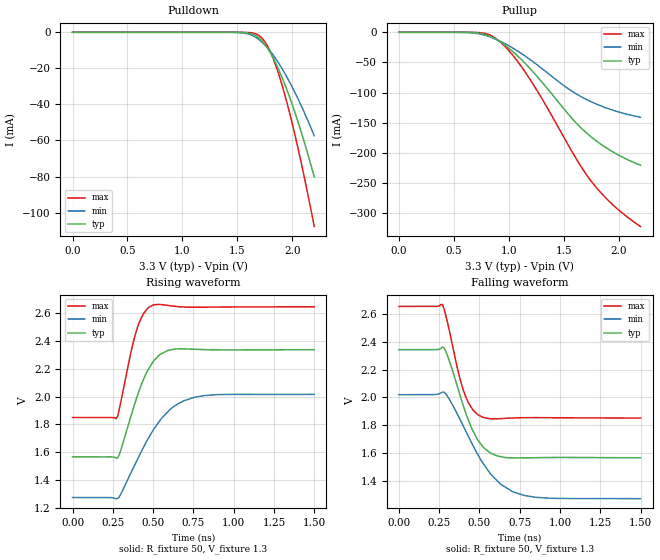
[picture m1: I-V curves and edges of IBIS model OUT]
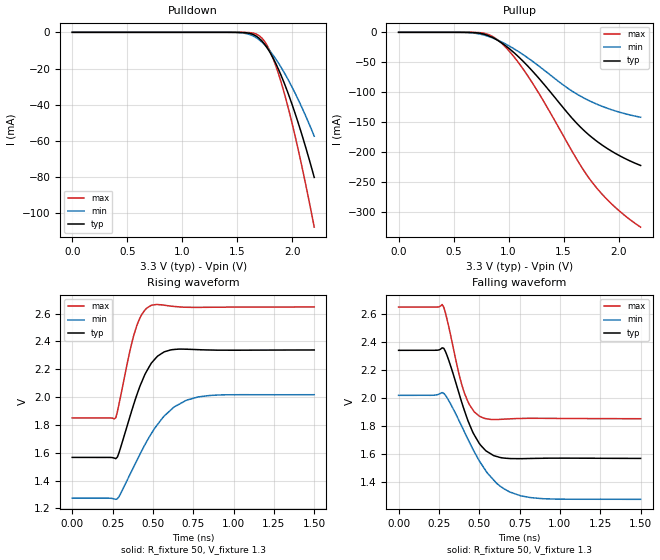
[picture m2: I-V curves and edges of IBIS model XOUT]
[IBIS Ver]   3.2
[Comment Char]   |_char
[File name]   vg7050efn_pecl.ibs
[File Rev]   1.0
[Date]   2019/07/25 5:42:03
[Source]
[Notes]
[Disclaimer]
Seiko Epson Corporation makes no warranty with respect to the information
contained herein.
[Copyright]
Copyright(C) 2016, Seiko Epson Corporation. All rights reserved.
[Component]   vg7050efn
Si_location Pin
Timing_location Pin
[Manufacturer]   Seiko Epson Corporation
[Package]
R_pkg   0.048   NA   NA
L_pkg   0.48n   NA   NA
C_pkg   0.21p   NA   NA
[Pin] signal_name   model_name   R_pin   L_pin   C_pin
1   VC   NC
2   OE   NC
3   GND   GND
4   OUT   OUT   0.043   4.00n   0.90p
5   XOUT   XOUT   0.028   4.00n   0.51p
6   VCC   POWER
[Diff Pin] inv_pin vdiff   tdelay_typ
4   5   0   0
| Models and submodels in the file (2): OUT (Output_ECL), XOUT (Output_ECL)
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[Model]   OUT
Model_type Output_ECL
Enable Active-High
Polarity Non-Inverting
Vref=1.3
Vmeas=1.97
Rref=50
Cref=0
C_comp   70f   70f   70f
[Temperature Range] 25   105   -40
[Voltage Range]   3.3   3.0   3.6
[Pullup Reference]  3.3   3.0   3.6
[Pulldown Reference]3.3   3.0   3.6
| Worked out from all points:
|   falling waveform, R_fixture 50, V_fixture 1.3: 20-80 % time 143ps typ, 225ps min, 102ps max; typ from 2.34 V to 1.57 V
|   rising waveform, R_fixture 50, V_fixture 1.3: 20-80 % time 137ps typ, 222ps min, 92ps max; typ from 1.57 V to 2.34 V
[Pullup]
0V        6.708pA    13.64pA    5.343pA
725mV     -1.244mA   -2.425mA   -398.1uA
825mV     -6.248mA   -7.358mA   -4.277mA
900mV     -13.34mA   -12.91mA   -12.59mA
1.025V    -30.17mA   -24.87mA   -35.5mA
1.175V    -56.49mA   -42.76mA   -72.92mA
1.325V    -87.53mA   -63.4mA    -117.2mA
1.575V    -142.7mA   -97.65mA   -197.7mA
1.675V    -161.6mA   -108.4mA   -227.6mA
1.75V     -173.5mA   -115.2mA   -246.9mA
1.95V     -198.6mA   -129.4mA   -286.6mA
2.2V      -220.6mA   -140.9mA   -322.3mA
[Pulldown]
0V        6.821pA    19.1pA     5.343pA
1.5V      -29.23uA   -130.7uA   -2.556uA
1.625V    -797.9uA   -1.484mA   -253.7uA
1.7V      -3.343mA   -4.169mA   -1.897mA
1.75V     -6.688mA   -6.98mA    -5.148mA
1.8V      -11.36mA   -10.53mA   -10.73mA
1.85V     -17.2mA    -14.73mA   -18.43mA
1.925V    -27.76mA   -22.06mA   -33.11mA
1.975V    -35.83mA   -27.57mA   -44.56mA
2.05V     -49.29mA   -36.64mA   -63.76mA
2.125V    -64.15mA   -46.62mA   -84.94mA
2.2V      -80.22mA   -57.41mA   -107.7mA
[Falling Waveform]
R_fixture=50
V_fixture=1.3
V_fixture_min=1.0
V_fixture_max=1.6
0s        2.342V     2.02V      2.651V
270ps     2.36V      2.038V     2.666V
310ps     2.272V     1.993V     2.494V
360ps     2.091V     1.888V     2.225V
400ps     1.941V     1.795V     2.052V
460ps     1.761V     1.656V     1.911V
520ps     1.65V      1.534V     1.859V
630ps     1.577V     1.381V     1.849V
780ps     1.568V     1.299V     1.856V
1.5ns     1.569V     1.276V     1.853V
[Rising Waveform]
R_fixture=50
V_fixture=1.3
V_fixture_min=1.0
V_fixture_max=1.6
0s        1.567V     1.274V     1.85V
270ps     1.559V     1.265V     1.842V
290ps     1.582V     1.278V     1.909V
370ps     1.889V     1.47V      2.36V
400ps     2V         1.542V     2.489V
440ps     2.123V     1.635V     2.598V
500ps     2.253V     1.759V     2.661V
620ps     2.34V      1.922V     2.653V
760ps     2.342V     1.997V     2.645V
1.5ns     2.339V     2.017V     2.648V
[Ramp]
R_load=50
dV/dt_r   4.649E-1/1.382E-10   4.469E-1/2.234E-10   4.805E-1/9.262E-11
dV/dt_f   4.649E-1/1.432E-10   4.469E-1/2.264E-10   4.805E-1/1.027E-10
|[End   OUT
[Model]   XOUT
Model_type Output_ECL
Enable Active-High
Polarity Inverting
Vref=1.3
Vmeas=1.97
Rref=50
Cref=0
C_comp   70f   70f   70f
[Temperature Range] 25   105   -40
[Voltage Range]   3.3   3.0   3.6
[Pullup Reference]  3.3   3.0   3.6
[Pulldown Reference]3.3   3.0   3.6
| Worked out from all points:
|   falling waveform, R_fixture 50, V_fixture 1.3: 20-80 % time 141ps typ, 220ps min, 102ps max; typ from 2.34 V to 1.57 V
|   rising waveform, R_fixture 50, V_fixture 1.3: 20-80 % time 139ps typ, 225ps min, 92.8ps max; typ from 1.57 V to 2.34 V
[Pullup]
0V        8.527pA    12.73pA    5.343pA
725mV     -1.243mA   -2.423mA   -397.5uA
825mV     -6.243mA   -7.353mA   -4.273mA
900mV     -13.33mA   -12.9mA    -12.57mA
1.025V    -30.15mA   -24.86mA   -35.47mA
1.175V    -56.46mA   -42.75mA   -72.86mA
1.325V    -87.5mA    -63.4mA    -117.2mA
1.55V     -137.6mA   -94.83mA   -189.8mA
1.65V     -157.6mA   -106.2mA   -221.1mA
1.75V     -174.3mA   -115.6mA   -248.1mA
1.95V     -199.9mA   -130.1mA   -288.9mA
2.2V      -222.3mA   -141.8mA   -325.3mA
[Pulldown]
0V        8.64pA     15.23pA    7.731pA
1.5V      -29.05uA   -130.1uA   -2.534uA
1.625V    -794.2uA   -1.479mA   -252.1uA
1.7V      -3.332mA   -4.158mA   -1.888mA
1.75V     -6.67mA    -6.966mA   -5.129mA
1.8V      -11.34mA   -10.52mA   -10.7mA
1.85V     -17.16mA   -14.71mA   -18.38mA
1.925V    -27.71mA   -22.04mA   -33.04mA
1.975V    -35.78mA   -27.53mA   -44.48mA
2.05V     -49.22mA   -36.61mA   -63.65mA
2.125V    -64.07mA   -46.58mA   -84.81mA
2.2V      -80.12mA   -57.36mA   -107.6mA
[Falling Waveform]
R_fixture=50
V_fixture=1.3
V_fixture_min=1.0
V_fixture_max=1.6
0s        2.342V     2.02V      2.651V
270ps     2.359V     2.039V     2.669V
310ps     2.273V     1.984V     2.515V
370ps     2.051V     1.85V      2.193V
410ps     1.904V     1.753V     2.029V
470ps     1.735V     1.614V     1.9V
510ps     1.661V     1.534V     1.866V
620ps     1.578V     1.379V     1.847V
760ps     1.567V     1.3V       1.854V
1.5ns     1.569V     1.276V     1.852V
[Rising Waveform]
R_fixture=50
V_fixture=1.3
V_fixture_min=1.0
V_fixture_max=1.6
0s        1.566V     1.274V     1.85V
270ps     1.558V     1.265V     1.851V
290ps     1.601V     1.285V     1.951V
360ps     1.869V     1.449V     2.345V
400ps     2.015V     1.544V     2.514V
450ps     2.162V     1.657V     2.625V
490ps     2.244V     1.737V     2.66V
630ps     2.342V     1.928V     2.652V
780ps     2.341V     2.001V     2.645V
1.5ns     2.339V     2.017V     2.648V
[Ramp]
R_load=50
dV/dt_r   4.648E-1/1.395E-10   4.469E-1/2.267E-10   4.802E-1/9.323E-11
dV/dt_f   4.648E-1/1.421E-10   4.469E-1/2.207E-10   4.802E-1/1.022E-10
|[End   XOUT
